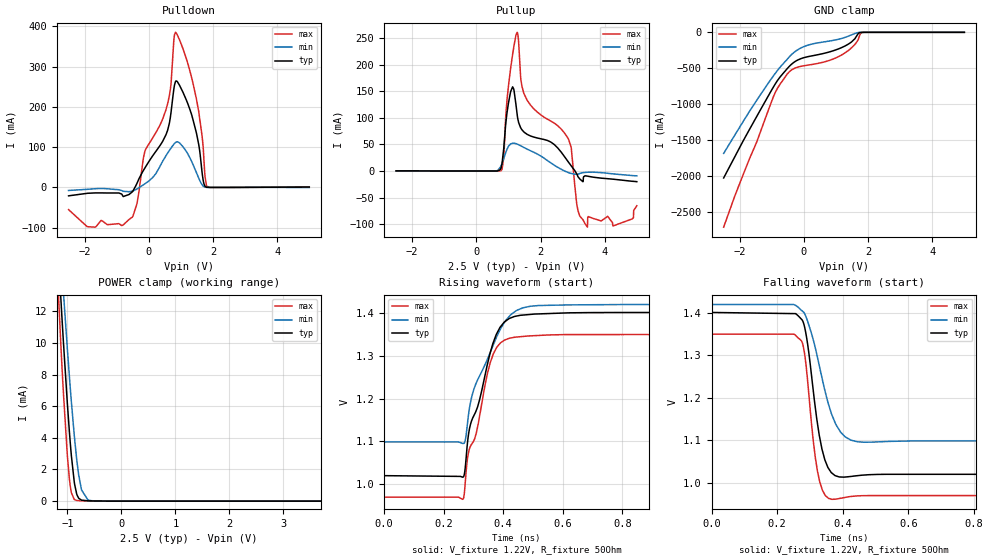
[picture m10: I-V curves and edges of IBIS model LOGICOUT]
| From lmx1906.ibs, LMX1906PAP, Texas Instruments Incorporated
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|   Model LOGICOUT
[Model]   LOGICOUT
Model_type   Output
Polarity   Non-Inverting
Vmeas = 1.25
Vref = 1.25
Cref = 2pF
Rref = 50
|   typ   min   max
C_comp   1.013pF   0.963pF   1.131pF
[Voltage Range]   2.5   2.4   2.6
[Temperature Range]   27   105   -40
[Pullup Reference]   2.5   2.4   2.6
[Pulldown Reference]   0   0   0
[Power Clamp Reference]   2.5   2.4   2.6
[GND Clamp Reference]   0   0   0
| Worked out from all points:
|   slope of the pulldown table from 0 to 0.375 V, typ, clamps not added: 8.7 ohm
|   slope of the pullup table from 0 to 0.375 V, typ, clamps not added: 83.3 kohm
|   POWER clamp passes 1 mA (typ) near -0.86 V on its own axis
|   falling waveform, V_fixture 1.22V, R_fixture 50Ohm: 20-80 % time 39.1ps typ, 62.3ps min, 30.6ps max; typ from 1.4 V to 1.02 V
|   rising waveform, V_fixture 1.22V, R_fixture 50Ohm: 20-80 % time 83.8ps typ, 102ps min, 75ps max; typ from 1.02 V to 1.4 V
[Pulldown]
|   Voltage   I(typ)   I(min)   I(max)
-2.5V     -20.84mA   -7.485mA   -55.02mA
-1.9V     -14.46mA   -4.603mA   -97.5mA
-512.5mV  -10.84mA   -9.304mA   -73.63mA
-362.5mV  11.37mA    -3.479mA   -37.56mA
-122.5mV  48.21mA    8.945mA    89.76mA
590mV     142.9mA    85.56mA    208.8mA
687.5mV   183.1mA    97.14mA    253.5mA
830mV     262.5mA    111.4mA    385mA
1.475V    138mA      38.56mA    222.9mA
1.7V      15.46mA    2.997mA    93.09mA
1.805V    422.5uA    196uA      3.068mA
5V        977.3uA    -150.9uA   1.293mA
[GND Clamp]
|   Voltage   I(typ)   I(min)   I(max)
-2.5V     -2.021A    -1.681A    -2.704A
-2.155V   -1.73A     -1.428A    -2.274A
-1.48V    -1.176A    -950.1mA   -1.533A
-940mV    -751.9mA   -598.4mA   -883.5mA
-752.5mV  -625.9mA   -489.6mA   -726.7mA
-407.5mV  -451.8mA   -318.5mA   -529.8mA
117.5mV   -338.8mA   -179.2mA   -455.6mA
1.115V    -223.4mA   -92.29mA   -329mA
1.587V    -89.54mA   -16.73mA   -169mA
1.7V      -15.4mA    -2.819mA   -93.09mA
1.805V    -416.1uA   -163.1uA   -3.067mA
5V        0A         0A         0A
[Pullup]
|   Voltage   I(typ)   I(min)   I(max)
-2.5V     313.5uA    12.66uA    391.5uA
770mV     5.682mA    9.946mA    800.5uA
852.5mV   41.96mA    23.46mA    24.25mA
920mV     91.58mA    35.42mA    106.5mA
1.07V     149.7mA    50.97mA    194mA
1.272V    106.1mA    50.73mA    261.1mA
1.393V    80.23mA    47.21mA    170.1mA
1.49V     73.07mA    44.08mA    144.8mA
2.877V    16.17mA    -3.181mA   59.16mA
3.23V     -15.28mA   -4.453mA   -85.39mA
4.265V    -15.36mA   -5.396mA   -103.3mA
5V        -20mA      -9.038mA   -65.28mA
[POWER Clamp]
|   Voltage   I(typ)   I(min)   I(max)
-2.5V     107.9mA    98.03mA    119.5mA
-1.292V   23.52mA    25.05mA    22.1mA
-1.113V   12.35mA    15.27mA    9.357mA
-1.075V   10.19mA    13.34mA    6.984mA
-1V       6.185mA    9.644mA    2.9mA
-962.5mV  4.409mA    7.906mA    1.425mA
-925mV    2.86mA     6.265mA    530uA
-865mV    1.062mA    3.912mA    90.81uA
-790mV    183.2uA    1.659mA    30.8uA
-737.5mV  61.23uA    707uA      23.43uA
-587.5mV  17.09uA    45.73uA    12.34uA
5V        0A         0A         0A
[Ramp]
R_load = 50
|   typ   min   max
dV/dt_r   0.228933/8.37698e-11   0.192928/1.02241e-10   0.228341/7.49914e-11
dV/dt_f   0.228933/3.91152e-11   0.192928/6.2259e-11   0.228341/3.05791e-11
[Falling Waveform]
V_fixture = 1.22V
V_fixture_min = 1.271V
V_fixture_max = 1.168V
R_fixture = 50Ohm
C_fixture = 0F
|   Time   V(typ)   V(min)   V(max)
0s        1.401V     1.42V      1.35V
273.9ps   1.385V     1.406V     1.334V
283.7ps   1.366V     1.398V     1.302V
293.2ps   1.324V     1.379V     1.236V
309.7ps   1.218V     1.337V     1.1V
322.9ps   1.139V     1.295V     1.026V
356.4ps   1.034V     1.185V     963.1mV
392.9ps   1.013V     1.119V     963.3mV
444.4ps   1.017V     1.096V     968.9mV
1.333ns   1.02V      1.099V     969.5mV
[Rising Waveform]
V_fixture = 1.22V
V_fixture_min = 1.271V
V_fixture_max = 1.168V
R_fixture = 50Ohm
C_fixture = 0F
|   Time   V(typ)   V(min)   V(max)
0s        1.02V      1.099V     969.5mV
266.1ps   1.017V     1.095V     965.8mV
273.8ps   1.048V     1.107V     1.015V
283.7ps   1.118V     1.164V     1.075V
309.7ps   1.173V     1.237V     1.12V
356.4ps   1.307V     1.308V     1.284V
404.3ps   1.379V     1.378V     1.337V
444.4ps   1.393V     1.406V     1.344V
518.5ps   1.398V     1.418V     1.348V
1.333ns   1.401V     1.42V      1.35V
